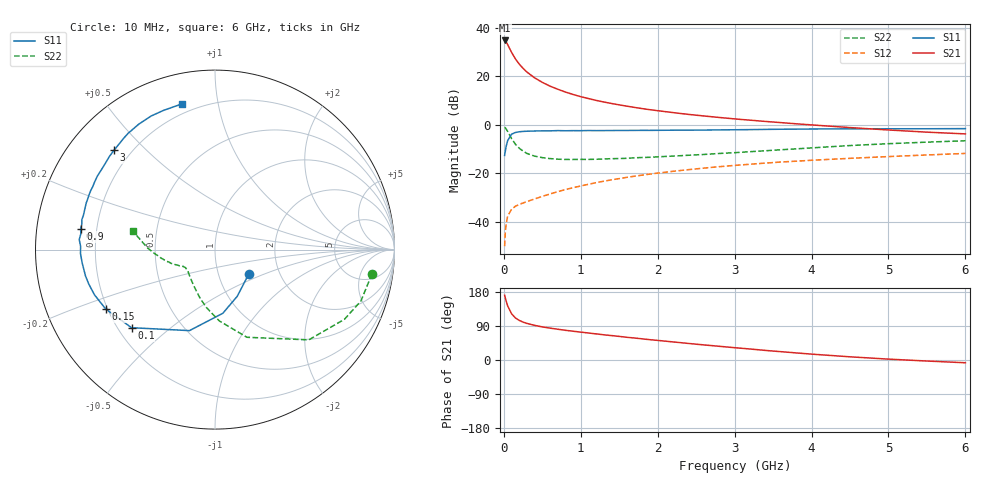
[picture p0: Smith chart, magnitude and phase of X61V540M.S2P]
! SIEMENS Small Signal Semiconductors
! BFP193W
! Si NPN RF Bipolar Junction Transistor in SOT343
! VCE = 1.5 V  IC = 40 mA
! Common Emitter S-Parameters:  April 1994
# GHz  S  MA  R  50
!  f  S11  S21  S12  S22
! GHz  MAG  ANG  MAG  ANG  MAG  ANG  MAG  ANG
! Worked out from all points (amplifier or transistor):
!   40 points, 10 MHz to 6 GHz, reference 50 ohm
!   highest |S21| = 34.9 dB at 10 MHz (marker M1)
!   |S21| within 3 dB of that: start of sweep to 69.85 MHz
!   unconditionally stable (mu >= 1): 553.1 MHz to 4.332 GHz
!   at 200 MHz: K = 0.57, MSG = 29.0 dB, |S12| = -32.9 dB
!   at 1.5 GHz: K = 1.17, MAG = 12.7 dB, |S12| = -22.2 dB
!   at 6 GHz: K = 0.97, MSG = 4.0 dB, |S12| = -11.8 dB
!   S11 on the Smith chart (normalised r, x): 10 MHz: 1.39, -0.41; 100 MHz: 0.25, -0.37; 150 MHz: 0.19, -0.25; 900 MHz: 0.14, +0.07; 3 GHz: 0.14, +0.40; 6 GHz: 0.15, +0.79
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0.01  0.2326 -36.5  55.28 170.8  0.0031 82.4  0.8851 -8.8
0.02  0.2884 -64.6  53.81 163.2  0.0063 73.3  0.8619 -19.4
0.03  0.3575 -83.0  51.52 155.6  0.0089 69.8  0.8191 -28.3
0.05  0.4733 -107.5  45.13 142.5  0.013 60.5  0.7252 -43.9
0.1  0.6369 -136.9  31.51 122.2  0.0179 46.9  0.5198 -70.0
0.15  0.693 -151.5  23.07 111.0  0.0207 41.9  0.3979 -86.6
0.2  0.7171 -159.4  17.94 104.5  0.0226 42.2  0.3278 -98.1
0.25  0.7289 -164.7  14.66 100.0  0.0242 43.7  0.2859 -106.5
0.3  0.7362 -168.4  12.29 96.6  0.0259 45.3  0.2555 -113.6
0.4  0.7435 -174.1  9.339 91.4  0.0293 48.6  0.225 -123.6
0.5  0.7498 -178.3  7.527 87.3  0.0332 52.0  0.2093 -130.8
0.6  0.7489 178.6  6.291 84.1  0.0371 54.3  0.2002 -136.2
0.8  0.7527 173.3  4.747 78.4  0.0458 58.1  0.1919 -142.7
0.9  0.7573 171.3  4.231 75.9  0.0501 59.0  0.192 -145.1
1.1  0.7603 167.3  3.485 71.2  0.059 60.5  0.1925 -148.4
1.6  0.7635 157.9  2.424 59.9  0.082 60.9  0.2029 -152.6
2.2  0.7729 148.0  1.785 47.7  0.1092 58.2  0.2254 -157.5
3  0.7892 135.5  1.322 32.5  0.1447 52.9  0.2652 -164.7
3.2  0.7944 132.5  1.246 29.0  0.1528 51.3  0.2779 -166.5
4.5  0.825 115.5  0.875 8.4  0.2026 41.4  0.3722 179.1
5.5  0.8277 106.8  0.704 -2.7  0.2379 34.5  0.4378 170.4
6  0.8327 102.6  0.648 -7.3  0.2559 31.5  0.4675 167.1
